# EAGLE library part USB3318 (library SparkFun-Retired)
Hi-speed USB transceiver Retired
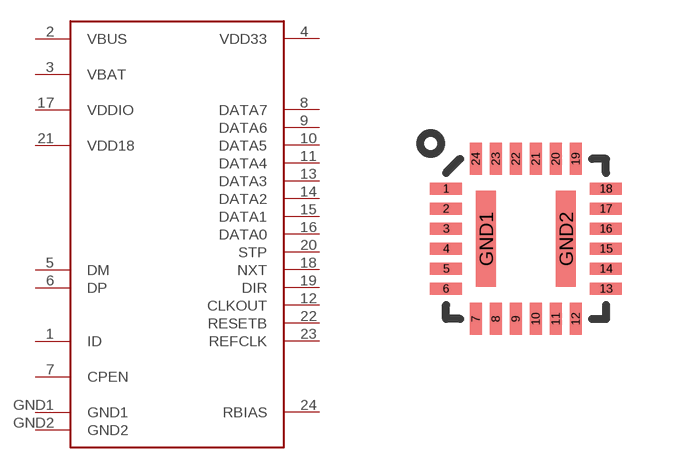
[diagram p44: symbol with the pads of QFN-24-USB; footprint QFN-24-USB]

Designator prefix -

## USB3318  [QFN-24-USB]
1  ID
2  VBUS
3  VBAT
4  VDD33
5  DM
6  DP
7  CPEN
8  DATA7
9  DATA6
10  DATA5
11  DATA4
12  CLKOUT
13  DATA3
14  DATA2
15  DATA1
16  DATA0
17  VDDIO
18  NXT
19  DIR
20  STP
21  VDD18
22  RESETB
23  REFCLK
24  RBIAS
GND1  GND1
GND2  GND2

## Footprint QFN-24-USB (pad centres in mm)
smd 0.8 x 0.3: 1 -2,1.25; 2 -2,0.75; 3 -2,0.25; 4 -2,-0.25; 5 -2,-0.75; 6 -2,-1.25; 13 2,-1.25; 14 2,-0.75; 15 2,-0.25; 16 2,0.25; 17 2,0.75; 18 2,1.25
smd 0.3 x 0.8: 7 -1.25,-2; 8 -0.75,-2; 9 -0.25,-2; 10 0.25,-2; 11 0.75,-2; 12 1.25,-2; 19 1.25,2; 20 0.75,2; 21 0.25,2; 22 -0.25,2; 23 -0.75,2; 24 -1.25,2
smd 0.5 x 2.4: GND1 -1,0; GND2 1,0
